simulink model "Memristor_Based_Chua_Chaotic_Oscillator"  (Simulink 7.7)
settings: Solver=ode113  StartTime=0  StopTime=1  RelTol=3e-14
libraries: fl_lib x7, nesl_utility x5, Memristor_lib x4, simulink x1

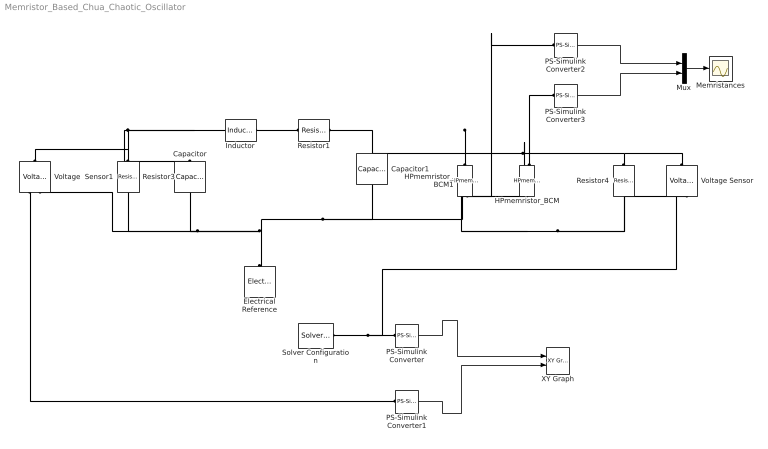
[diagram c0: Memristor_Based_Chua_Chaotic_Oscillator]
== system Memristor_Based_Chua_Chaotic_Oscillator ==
  Capacitor : fl_lib/Electrical/Electrical Elements/Capacitor  SystemSampleTime=-1  c=37e-9 F  v0=0.02 V  r=0 Ohm  g=0 1/Ohm  i_Log=off  v_Log=off  vc_Log=off  LocalVarNames=|i|v|vc  LocalVarDescs=|i|v|Internal variable for voltage across capacitor term  LocalVarLogging=[0 0 0]
  Capacitor1 : fl_lib/Electrical/Electrical Elements/Capacitor  SystemSampleTime=-1  c=50e-9 F  v0=0.006 V  r=0 Ohm  g=0 1/Ohm  i_Log=off  v_Log=off  vc_Log=off  LocalVarNames=|i|v|vc  LocalVarDescs=|i|v|Internal variable for voltage across capacitor term  LocalVarLogging=[0 0 0]
  Electrical Reference : fl_lib/Electrical/Electrical Elements/Electrical Reference  SystemSampleTime=-1  i_Log=off  LocalVarNames=|i  LocalVarDescs=|i  LocalVarLogging=0
  HPmemristor_BCM : Memristor_lib/HPmemristor_BCM  SystemSampleTime=-1  G_off=6e-5 1/Ohm  G_on=0.0019 1/Ohm  N=1 1/Ohm  u_v=1e-11 m^2/s/V  D=1e-8 m  x0=0 Ohm  t0=1.1212e-005 s  i0=1 A  VT1=0 V  VT0=0 V  i_Log=off  v_Log=off  x_Log=off  F_Log=off  W_Log=off  LocalVarNames=|i|v|x|F|W  LocalVarDescs=|i|v|x|F|W  LocalVarLogging=[0 0 0 0 0]
  HPmemristor_BCM1 : Memristor_lib/HPmemristor_BCM  SystemSampleTime=-1  G_off=6e-5 1/Ohm  G_on=0.0019 1/Ohm  N=1 1/Ohm  u_v=1e-11 m^2/s/V  D=1e-8 m  x0=0 Ohm  t0=1.12e-5 s  i0=1 A  VT1=0 V  VT0=0 V  i_Log=off  v_Log=off  x_Log=off  F_Log=off  W_Log=off  LocalVarNames=|i|v|x|F|W  LocalVarDescs=|i|v|x|F|W  LocalVarLogging=[0 0 0 0 0]
  Inductor : fl_lib/Electrical/Electrical Elements/Inductor  SystemSampleTime=-1  l=100e-3 H  i0=.99e-3 A  r=0 Ohm  g=0 1/Ohm  i_Log=off  v_Log=off  i_L_Log=off  LocalVarNames=|i|v|i_L  LocalVarDescs=|i|v|Internal variable for current through inductor term  LocalVarLogging=[0 0 0]
  Memristances : Scope
  Mux : Mux  Inputs=2
  PS-Simulink Converter{,1..3} (4 alike) : nesl_utility/PS-Simulink Converter  SystemSampleTime=-1  PhysicalDomain=network_engine_domain  LeftPortType=input  RightPortType=output  SubClassName=ps_output  Unit=1  AffineConversion=off
  Resistor1 : fl_lib/Electrical/Electrical Elements/Resistor  SystemSampleTime=-1  R=303.030303 Ohm  i_Log=off  v_Log=off  LocalVarNames=|i|v  LocalVarDescs=|i|v  LocalVarLogging=[0 0]
  Resistor3 : Memristor_lib/Other Components/Resistor  SystemSampleTime=-1  R=-2500 Ohm  i_Log=off  v_Log=off  LocalVarNames=|i|v  LocalVarDescs=|i|v  LocalVarLogging=[0 0]
  Resistor4 : Memristor_lib/Other Components/Resistor  SystemSampleTime=-1  R=-263504.6113 Ohm  i_Log=off  v_Log=off  LocalVarNames=|i|v  LocalVarDescs=|i|v  LocalVarLogging=[0 0]
  Solver Configuration : nesl_utility/Solver Configuration  SystemSampleTime=-1  PhysicalDomain=network_engine_domain  LeftPortType=input  RightPortType=generic  SubClassName=solver  Accelerate=off  Profile=off  ResidualTolerance=1e-9  MaxNonlinIter=3  MaxModeIter=2  DoFixedCost=off  UseLocalSampling=off  DoDC=off  LinearAlgebra=Sparse  LocalSolverSampleTime=.001  LocalSolverChoice=NE_BACKWARD_EULER_ADVANCER  UseLocalSolver=off
  Voltage  Sensor1 : fl_lib/Electrical/Electrical Sensors/Voltage Sensor  SystemSampleTime=-1  i1_Log=off  v1_Log=off  LocalVarNames=|i1|v1  LocalVarDescs=|i1|v1  LocalVarLogging=[0 0]
  Voltage Sensor : fl_lib/Electrical/Electrical Sensors/Voltage Sensor  SystemSampleTime=-1  i1_Log=off  v1_Log=off  LocalVarNames=|i1|v1  LocalVarDescs=|i1|v1  LocalVarLogging=[0 0]
  XY Graph : simulink/Sinks/XY Graph  SystemSampleTime=-1  xmin=-2e5  xmax=2e5  ymin=-2e5  ymax=2e5  st=-1
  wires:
  PS-Simulink Converter1/1 -> XY Graph/2
  PS-Simulink Converter/1 -> XY Graph/1
  Mux/1 -> Memristances/1
  PS-Simulink Converter2/1 -> Mux/1
  PS-Simulink Converter3/1 -> Mux/2
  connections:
  HPmemristor_BCM1/LConn1 -- HPmemristor_BCM/RConn1 -- Voltage Sensor/LConn1 -- Resistor4/LConn1 -- Resistor1/RConn1 -- Capacitor1/LConn1
  HPmemristor_BCM1/RConn1 -- Voltage Sensor/RConn2 -- Resistor4/RConn1 -- HPmemristor_BCM/LConn1 -- Capacitor1/RConn1 -- Electrical Reference/LConn1 -- Capacitor/RConn1 -- Voltage  Sensor1/RConn2 -- Resistor3/RConn1
  Solver Configuration/RConn1 -- PS-Simulink Converter/LConn1 -- Voltage Sensor/RConn1
  Resistor3/LConn1 -- Inductor/LConn1 -- Capacitor/LConn1 -- Voltage  Sensor1/LConn1
  Inductor/RConn1 -- Resistor1/LConn1
  Voltage  Sensor1/RConn1 -- PS-Simulink Converter1/LConn1
  HPmemristor_BCM1/RConn2 -- PS-Simulink Converter2/LConn1
  HPmemristor_BCM/RConn2 -- PS-Simulink Converter3/LConn1
